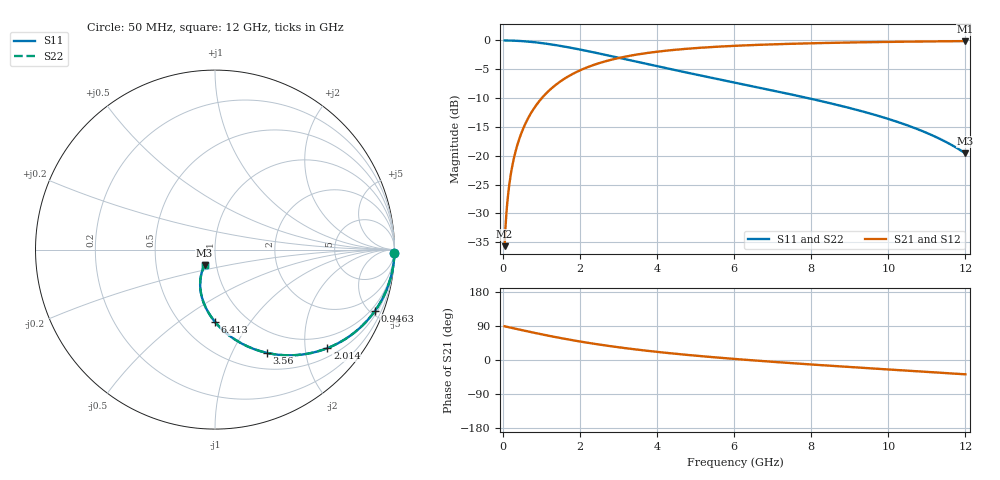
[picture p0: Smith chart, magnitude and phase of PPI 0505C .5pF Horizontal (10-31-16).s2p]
# MHz S MA R 50
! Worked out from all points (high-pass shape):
!   1601 points, 50 MHz to 12 GHz, reference 50 ohm
!   highest |S21| = -0.12 dB at 12 GHz (marker M1); lowest = -35.7 dB at 50 MHz (marker M2)
!   |S21| within 3 dB of the highest: 2.963 GHz to end of sweep
!   lowest |S11| = -19.6 dB at 12 GHz (marker M3), VSWR 1.23, Z = 43.9 - j7.7 ohm
!   |S11| at or under -10 dB: 7.912 GHz to end of sweep
!   |S22| runs from -19.6 to 0.0 dB; largest |S21 - S12| = 0
!   S11 on the Smith chart (normalised r, x): 50 MHz: open; 946.2 MHz: 0.69, -5.34; 2.014 GHz: 0.70, -2.49; 3.56 GHz: 0.70, -1.38; 6.413 GHz: 0.72, -0.70; 12 GHz: 0.88, -0.15
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50  0.9999 -1.1  0.0164 88.9  0.0164 88.9  0.9999 -1.1
79.875  0.9997 -1.8  0.0262 88.2  0.0262 88.2  0.9997 -1.8
139.625  0.9989 -3.2  0.04577 86.8  0.04577 86.8  0.9989 -3.2
176.9688  0.9983 -4.0  0.05797 86.0  0.05797 86.0  0.9983 -4.0
244.1875  0.9968 -5.5  0.07987 84.5  0.07987 84.5  0.9968 -5.5
333.8125  0.994 -7.5  0.1089 82.5  0.1089 82.5  0.994 -7.5
445.8438  0.9894 -10.0  0.1448 79.9  0.1448 79.9  0.9894 -10.0
587.75  0.9818 -13.2  0.1894 76.8  0.1894 76.8  0.9818 -13.2
946.25  0.9547 -20.9  0.2966 69.1  0.2966 69.1  0.9547 -20.9
1416.781  0.9061 -30.4  0.4218 59.5  0.4218 59.5  0.9061 -30.4
2014.281  0.8327 -41.2  0.552 48.7  0.552 48.7  0.8327 -41.2
2044.156  0.8289 -41.7  0.5577 48.2  0.5577 48.2  0.8289 -41.7
2723.812  0.7425 -52.3  0.6676 37.5  0.6676 37.5  0.7425 -52.3
3560.312  0.6444 -63.3  0.7619 26.5  0.7619 26.5  0.6444 -63.3
4038.312  0.5945 -68.7  0.801 21.1  0.801 21.1  0.5945 -68.7
4971.906  0.5095 -77.9  0.8568 11.7  0.8568 11.7  0.5095 -77.9
6025  0.4303 -86.8  0.8985 2.7  0.8985 2.7  0.4303 -86.8
6413.375  0.4044 -89.8  0.9102 -0.4  0.9102 -0.4  0.4044 -89.8
8019.156  0.3104 -101.1  0.9453 -12.0  0.9453 -12.0  0.3104 -101.1
10013.31  0.2078 -113.5  0.9718 -25.1  0.9718 -25.1  0.2078 -113.5
11103.75  0.1522 -119.6  0.9812 -32.0  0.9812 -32.0  0.1522 -119.6
12000  0.1046 -123.9  0.9868 -37.8  0.9868 -37.8  0.1046 -123.9
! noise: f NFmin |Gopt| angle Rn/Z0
50  0.001875  0.9838  1.054  0.0264
1372  0.005899  0.7842  9.374  0.005578
2701  0.0091  0.7223  13.9  0.006405
4031  0.01196  0.6884  18.45  0.007276
5360  0.01466  0.667  22.99  0.008127
6682  0.01728  0.6533  27.46  0.008977
8012  0.01992  0.645  31.87  0.009861
9341  0.0226  0.641  36.17  0.0108
1.067e+04  0.02537  0.6407  40.34  0.01183
1.2e+04  0.02828  0.6434  44.38  0.01297
